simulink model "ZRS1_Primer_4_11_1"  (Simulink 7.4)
settings: Solver=ode45  StartTime=0.0  StopTime=30  MaxStep=1  RelTol=1e-5
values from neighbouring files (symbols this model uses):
  k = 2    [basic_control.m]    (also in basic_control_1.m; ZRS1_Primer4_11.m = 0.7; ZRS1_Primer4_11_1.m = 0.7; ZRS2_primer_2_13.m = 100)

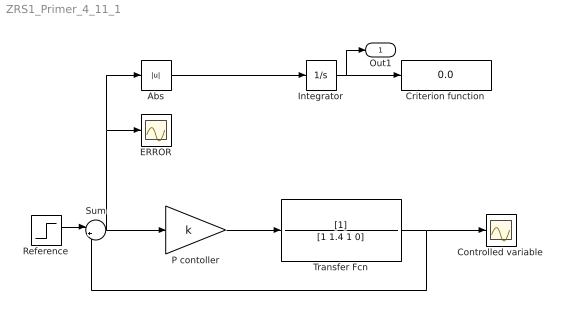
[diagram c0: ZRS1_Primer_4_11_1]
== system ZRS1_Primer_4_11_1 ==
  Abs : Abs
  Controlled variable : Scope
  Criterion function : Display
  ERROR : Scope
  Integrator : Integrator
  P contoller : Gain  Gain=k  ParameterDataType=sfix(16)  ParameterScaling=2^0  OutDataType=sfix(16)  OutScaling=2^0
  Reference : Step  Time=0  SampleTime=0
  Sum : Sum  Inputs=|+-  OutDataType=sfix(16)  OutScaling=2^0
  Transfer Fcn : TransferFcn  Denominator=[1 1.4 1 0]
  Out1 : Outport  OutDataType=sfix(16)  OutScaling=2^0
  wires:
  Reference/1 -> Sum/1
  Sum/1 -> ERROR/1, Abs/1, P contoller/1
  Integrator/1 -> Criterion function/1, Out1/1
  Transfer Fcn/1 -> Controlled variable/1, Sum/2
  P contoller/1 -> Transfer Fcn/1
  Abs/1 -> Integrator/1
